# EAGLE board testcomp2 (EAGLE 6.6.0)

Size 100 x 80 mm. Coordinates in mm from the lower left corner, seen from the top.
Outline: 0,0 100,0 100,80 0,80 0,0
Copper layers (1*16): Top 0.035mm / dielectric 1.5mm / Bottom 0.035mm
Design rules "Fusion_eagle_rule_v1.1": minimum track width 6mil, minimum drill 12mil, track to track 6mil, track to pad 6mil, pad to pad 6mil, via to via 6mil, smd to smd 0mil, copper to edge 10mil, drill to drill 10mil, minimum pad ring 10mil, minimum via ring 6mil, stop-mask expansion 2mil, vias tented up to drill 100mil, thermal gap 10mil

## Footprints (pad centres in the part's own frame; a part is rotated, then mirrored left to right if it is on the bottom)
C0805 = smd 1.3 x 1.5: 1 -0.95,0; 2 0.95,0
SOT23 = smd 1 x 1.4: 1 -0.95,-1.1; 2 0.95,-1.1; 3 0,1.354
R0805 = smd 1.3 x 1.5: 1 -0.95,0; 2 0.95,0

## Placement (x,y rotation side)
C1  100nF  [C0805]  6.44,10.71 270 top
C2  100nF  [C0805]  5.56,6.29 90 top
C3  100nF  [C0805]  13.56,6.29 90 top
C4  100nF  [C0805]  14.44,10.71 270 top
C5  100nF  [C0805]  21.56,6.29 90 top
C6  100nF  [C0805]  22.44,10.71 270 top
C7  100nF  [C0805]  29.56,6.29 90 top
C8  100nF  [C0805]  30.44,10.71 270 top
C9  100nF  [C0805]  37.56,6.29 90 top
C10  100nF  [C0805]  38.44,10.71 270 top
C11  100nF  [C0805]  45.56,6.29 90 top
C12  100nF  [C0805]  46.44,10.71 270 top
C13  100nF  [C0805]  53.56,6.29 90 top
C14  100nF  [C0805]  54.44,10.71 270 top
C15  100nF  [C0805]  61.56,6.29 90 top
C16  100nF  [C0805]  62.44,10.71 270 top
C17  100nF  [C0805]  69.56,6.29 90 top
C18  100nF  [C0805]  70.44,10.71 270 top
C19  100nF  [C0805]  77.56,6.29 90 top
C20  100nF  [C0805]  78.44,10.71 270 top
C21  100nF  [C0805]  85.56,6.29 90 top
C22  100nF  [C0805]  86.44,10.71 270 top
C23  100nF  [C0805]  93.56,6.29 90 top
C24  100nF  [C0805]  94.44,10.71 270 top
C25  100nF  [C0805]  5.56,15.29 90 top
C26  100nF  [C0805]  6.44,19.71 270 top
C27  100nF  [C0805]  13.56,15.29 90 top
C28  100nF  [C0805]  14.44,19.71 270 top
C29  100nF  [C0805]  21.56,15.29 90 top
C30  100nF  [C0805]  22.44,19.71 270 top
C31  100nF  [C0805]  29.56,15.29 90 top
C32  100nF  [C0805]  30.44,19.71 270 top
C33  100nF  [C0805]  37.56,15.29 90 top
C34  100nF  [C0805]  38.44,19.71 270 top
C35  100nF  [C0805]  45.56,15.29 90 top
C36  100nF  [C0805]  46.44,19.71 270 top
C37  100nF  [C0805]  53.56,15.29 90 top
C38  100nF  [C0805]  54.44,19.71 270 top
C39  100nF  [C0805]  61.56,15.29 90 top
C40  100nF  [C0805]  62.44,19.71 270 top
C41  100nF  [C0805]  69.56,15.29 90 top
C42  100nF  [C0805]  70.44,19.71 270 top
C43  100nF  [C0805]  77.56,15.29 90 top
C44  100nF  [C0805]  78.44,19.71 270 top
C45  100nF  [C0805]  85.56,15.29 90 top
C46  100nF  [C0805]  86.44,19.71 270 top
C47  100nF  [C0805]  93.56,15.29 90 top
C48  100nF  [C0805]  94.44,19.71 270 top
C49  100nF  [C0805]  5.56,24.29 90 top
C50  100nF  [C0805]  6.44,28.71 270 top
C51  100nF  [C0805]  13.56,24.29 90 top
C52  100nF  [C0805]  14.44,28.71 270 top
C53  100nF  [C0805]  21.56,24.29 90 top
C54  100nF  [C0805]  22.44,28.71 270 top
C55  100nF  [C0805]  29.56,24.29 90 top
C56  100nF  [C0805]  30.44,28.71 270 top
C57  100nF  [C0805]  37.56,24.29 90 top
C58  100nF  [C0805]  38.44,28.71 270 top
C59  100nF  [C0805]  45.56,24.29 90 top
C60  100nF  [C0805]  46.44,28.71 270 top
C61  100nF  [C0805]  53.56,24.29 90 top
C62  100nF  [C0805]  54.44,28.71 270 top
C63  100nF  [C0805]  61.56,24.29 90 top
C64  100nF  [C0805]  62.44,28.71 270 top
C65  100nF  [C0805]  69.56,24.29 90 top
C66  100nF  [C0805]  70.44,28.71 270 top
C67  100nF  [C0805]  77.56,24.29 90 top
C68  100nF  [C0805]  78.44,28.71 270 top
C69  100nF  [C0805]  85.56,24.29 90 top
C70  100nF  [C0805]  86.44,28.71 270 top
C71  100nF  [C0805]  93.56,24.29 90 top
C72  100nF  [C0805]  94.44,28.71 270 top
C73  100nF  [C0805]  5.56,33.29 90 top
C74  100nF  [C0805]  6.44,37.71 270 top
C75  100nF  [C0805]  13.56,33.29 90 top
C76  100nF  [C0805]  14.44,37.71 270 top
C77  100nF  [C0805]  21.56,33.29 90 top
C78  100nF  [C0805]  22.44,37.71 270 top
C79  100nF  [C0805]  29.56,33.29 90 top
C80  100nF  [C0805]  30.44,37.71 270 top
C81  100nF  [C0805]  37.56,33.29 90 top
C82  100nF  [C0805]  38.44,37.71 270 top
C83  100nF  [C0805]  45.56,33.29 90 top
C84  100nF  [C0805]  46.44,37.71 270 top
C85  100nF  [C0805]  53.56,33.29 90 top
C86  100nF  [C0805]  54.44,37.71 270 top
C87  100nF  [C0805]  61.56,33.29 90 top
C88  100nF  [C0805]  62.44,37.71 270 top
C89  100nF  [C0805]  69.56,33.29 90 top
C90  100nF  [C0805]  70.44,37.71 270 top
C91  100nF  [C0805]  77.56,33.29 90 top
C92  100nF  [C0805]  78.44,37.71 270 top
C93  100nF  [C0805]  85.56,33.29 90 top
C94  100nF  [C0805]  86.44,37.71 270 top
C95  100nF  [C0805]  93.56,33.29 90 top
C96  100nF  [C0805]  94.44,37.71 270 top
C97  100nF  [C0805]  5.56,42.29 90 top
C98  100nF  [C0805]  6.44,46.71 270 top
C99  100nF  [C0805]  13.56,42.29 90 top
C100  100nF  [C0805]  14.44,46.71 270 top
C101  100nF  [C0805]  21.56,42.29 90 top
C102  100nF  [C0805]  22.44,46.71 270 top
C103  100nF  [C0805]  29.56,42.29 90 top
C104  100nF  [C0805]  30.44,46.71 270 top
C105  100nF  [C0805]  37.56,42.29 90 top
C106  100nF  [C0805]  38.44,46.71 270 top
C107  100nF  [C0805]  45.56,42.29 90 top
C108  100nF  [C0805]  46.44,46.71 270 top
C109  100nF  [C0805]  53.56,42.29 90 top
C110  100nF  [C0805]  54.44,46.71 270 top
C111  100nF  [C0805]  61.56,42.29 90 top
C112  100nF  [C0805]  62.44,46.71 270 top
C113  100nF  [C0805]  69.56,42.29 90 top
C114  100nF  [C0805]  70.44,46.71 270 top
C115  100nF  [C0805]  77.56,42.29 90 top
C116  100nF  [C0805]  78.44,46.71 270 top
C117  100nF  [C0805]  85.56,42.29 90 top
C118  100nF  [C0805]  86.44,46.71 270 top
C119  100nF  [C0805]  93.56,42.29 90 top
C120  100nF  [C0805]  94.44,46.71 270 top
C121  100nF  [C0805]  5.56,51.29 90 top
C122  100nF  [C0805]  6.44,55.71 270 top
C123  100nF  [C0805]  13.56,51.29 90 top
C124  100nF  [C0805]  14.44,55.71 270 top
C125  100nF  [C0805]  21.56,51.29 90 top
C126  100nF  [C0805]  22.44,55.71 270 top
C127  100nF  [C0805]  29.56,51.29 90 top
C128  100nF  [C0805]  30.44,55.71 270 top
C129  100nF  [C0805]  37.56,51.29 90 top
C130  100nF  [C0805]  38.44,55.71 270 top
C131  100nF  [C0805]  45.56,51.29 90 top
C132  100nF  [C0805]  46.44,55.71 270 top
C133  100nF  [C0805]  53.56,51.29 90 top
C134  100nF  [C0805]  54.44,55.71 270 top
C135  100nF  [C0805]  61.56,51.29 90 top
C136  100nF  [C0805]  62.44,55.71 270 top
C137  100nF  [C0805]  69.56,51.29 90 top
C138  100nF  [C0805]  70.44,55.71 270 top
C139  100nF  [C0805]  77.56,51.29 90 top
C140  100nF  [C0805]  78.44,55.71 270 top
C141  100nF  [C0805]  85.56,51.29 90 top
C142  100nF  [C0805]  86.44,55.71 270 top
C143  100nF  [C0805]  93.56,51.29 90 top
C144  100nF  [C0805]  94.44,55.71 270 top
C145  100nF  [C0805]  5.56,60.29 90 top
C146  100nF  [C0805]  6.44,64.71 270 top
C147  100nF  [C0805]  13.56,60.29 90 top
C148  100nF  [C0805]  14.44,64.71 270 top
C149  100nF  [C0805]  21.56,60.29 90 top
C150  100nF  [C0805]  22.44,64.71 270 top
C151  100nF  [C0805]  29.56,60.29 90 top
C152  100nF  [C0805]  30.44,64.71 270 top
C153  100nF  [C0805]  37.56,60.29 90 top
C154  100nF  [C0805]  38.44,64.71 270 top
C155  100nF  [C0805]  45.56,60.29 90 top
C156  100nF  [C0805]  46.44,64.71 270 top
C157  100nF  [C0805]  53.56,60.29 90 top
C158  100nF  [C0805]  54.44,64.71 270 top
C159  100nF  [C0805]  61.56,60.29 90 top
C160  100nF  [C0805]  62.44,64.71 270 top
C161  100nF  [C0805]  69.56,60.29 90 top
C162  100nF  [C0805]  70.44,64.71 270 top
C163  100nF  [C0805]  77.56,60.29 90 top
C164  100nF  [C0805]  78.44,64.71 270 top
C165  100nF  [C0805]  85.56,60.29 90 top
C166  100nF  [C0805]  86.44,64.71 270 top
C167  100nF  [C0805]  93.56,60.29 90 top
C168  100nF  [C0805]  94.44,64.71 270 top
C169  100nF  [C0805]  5.56,69.29 90 top
C170  100nF  [C0805]  6.44,73.71 270 top
C171  100nF  [C0805]  13.56,69.29 90 top
C172  100nF  [C0805]  14.44,73.71 270 top
C173  100nF  [C0805]  21.56,69.29 90 top
C174  100nF  [C0805]  22.44,73.71 270 top
C175  100nF  [C0805]  29.56,69.29 90 top
C176  100nF  [C0805]  30.44,73.71 270 top
C177  100nF  [C0805]  37.56,69.29 90 top
C178  100nF  [C0805]  38.44,73.71 270 top
C179  100nF  [C0805]  45.56,69.29 90 top
C180  100nF  [C0805]  46.44,73.71 270 top
C181  100nF  [C0805]  53.56,69.29 90 top
C182  100nF  [C0805]  54.44,73.71 270 top
C183  100nF  [C0805]  61.56,69.29 90 top
C184  100nF  [C0805]  62.44,73.71 270 top
C185  100nF  [C0805]  69.56,69.29 90 top
C186  100nF  [C0805]  70.44,73.71 270 top
C187  100nF  [C0805]  77.56,69.29 90 top
C188  100nF  [C0805]  78.44,73.71 270 top
C189  100nF  [C0805]  85.56,69.29 90 top
C190  100nF  [C0805]  86.44,73.71 270 top
C191  100nF  [C0805]  93.56,69.29 90 top
C192  100nF  [C0805]  94.44,73.71 270 top
D1  BAT54C  [SOT23]  3.78,10.35 0 top
D2  BAT54C  [SOT23]  8.22,6.65 180 top
D3  BAT54C  [SOT23]  11.78,10.35 0 top
D4  BAT54C  [SOT23]  16.22,6.65 180 top
D5  BAT54C  [SOT23]  19.78,10.35 0 top
D6  BAT54C  [SOT23]  24.22,6.65 180 top
D7  BAT54C  [SOT23]  27.78,10.35 0 top
D8  BAT54C  [SOT23]  32.22,6.65 180 top
D9  BAT54C  [SOT23]  35.78,10.35 0 top
D10  BAT54C  [SOT23]  40.22,6.65 180 top
D11  BAT54C  [SOT23]  43.78,10.35 0 top
D12  BAT54C  [SOT23]  48.22,6.65 180 top
D13  BAT54C  [SOT23]  51.78,10.35 0 top
D14  BAT54C  [SOT23]  56.22,6.65 180 top
D15  BAT54C  [SOT23]  59.78,10.35 0 top
D16  BAT54C  [SOT23]  64.22,6.65 180 top
D17  BAT54C  [SOT23]  67.78,10.35 0 top
D18  BAT54C  [SOT23]  72.22,6.65 180 top
D19  BAT54C  [SOT23]  75.78,10.35 0 top
D20  BAT54C  [SOT23]  80.22,6.65 180 top
D21  BAT54C  [SOT23]  83.78,10.35 0 top
D22  BAT54C  [SOT23]  88.22,6.65 180 top
D23  BAT54C  [SOT23]  91.78,10.35 0 top
D24  BAT54C  [SOT23]  96.22,6.65 180 top
D25  BAT54C  [SOT23]  3.78,19.35 0 top
D26  BAT54C  [SOT23]  8.22,15.65 180 top
D27  BAT54C  [SOT23]  11.78,19.35 0 top
D28  BAT54C  [SOT23]  16.22,15.65 180 top
D29  BAT54C  [SOT23]  19.78,19.35 0 top
D30  BAT54C  [SOT23]  24.22,15.65 180 top
D31  BAT54C  [SOT23]  27.78,19.35 0 top
D32  BAT54C  [SOT23]  32.22,15.65 180 top
D33  BAT54C  [SOT23]  35.78,19.35 0 top
D34  BAT54C  [SOT23]  40.22,15.65 180 top
D35  BAT54C  [SOT23]  43.78,19.35 0 top
D36  BAT54C  [SOT23]  48.22,15.65 180 top
D37  BAT54C  [SOT23]  51.78,19.35 0 top
D38  BAT54C  [SOT23]  56.22,15.65 180 top
D39  BAT54C  [SOT23]  59.78,19.35 0 top
D40  BAT54C  [SOT23]  64.22,15.65 180 top
D41  BAT54C  [SOT23]  67.78,19.35 0 top
D42  BAT54C  [SOT23]  72.22,15.65 180 top
D43  BAT54C  [SOT23]  75.78,19.35 0 top
D44  BAT54C  [SOT23]  80.22,15.65 180 top
D45  BAT54C  [SOT23]  83.78,19.35 0 top
D46  BAT54C  [SOT23]  88.22,15.65 180 top
D47  BAT54C  [SOT23]  91.78,19.35 0 top
D48  BAT54C  [SOT23]  96.22,15.65 180 top
D49  BAT54C  [SOT23]  3.78,28.35 0 top
D50  BAT54C  [SOT23]  8.22,24.65 180 top
D51  BAT54C  [SOT23]  11.78,28.35 0 top
D52  BAT54C  [SOT23]  16.22,24.65 180 top
D53  BAT54C  [SOT23]  19.78,28.35 0 top
D54  BAT54C  [SOT23]  24.22,24.65 180 top
D55  BAT54C  [SOT23]  27.78,28.35 0 top
D56  BAT54C  [SOT23]  32.22,24.65 180 top
D57  BAT54C  [SOT23]  35.78,28.35 0 top
D58  BAT54C  [SOT23]  40.22,24.65 180 top
D59  BAT54C  [SOT23]  43.78,28.35 0 top
D60  BAT54C  [SOT23]  48.22,24.65 180 top
D61  BAT54C  [SOT23]  51.78,28.35 0 top
D62  BAT54C  [SOT23]  56.22,24.65 180 top
D63  BAT54C  [SOT23]  59.78,28.35 0 top
D64  BAT54C  [SOT23]  64.22,24.65 180 top
D65  BAT54C  [SOT23]  67.78,28.35 0 top
D66  BAT54C  [SOT23]  72.22,24.65 180 top
D67  BAT54C  [SOT23]  75.78,28.35 0 top
D68  BAT54C  [SOT23]  80.22,24.65 180 top
D69  BAT54C  [SOT23]  83.78,28.35 0 top
D70  BAT54C  [SOT23]  88.22,24.65 180 top
D71  BAT54C  [SOT23]  91.78,28.35 0 top
D72  BAT54C  [SOT23]  96.22,24.65 180 top
D73  BAT54C  [SOT23]  3.78,37.35 0 top
D74  BAT54C  [SOT23]  8.22,33.65 180 top
D75  BAT54C  [SOT23]  11.78,37.35 0 top
D76  BAT54C  [SOT23]  16.22,33.65 180 top
D77  BAT54C  [SOT23]  19.78,37.35 0 top
D78  BAT54C  [SOT23]  24.22,33.65 180 top
D79  BAT54C  [SOT23]  27.78,37.35 0 top
D80  BAT54C  [SOT23]  32.22,33.65 180 top
D81  BAT54C  [SOT23]  35.78,37.35 0 top
D82  BAT54C  [SOT23]  40.22,33.65 180 top
D83  BAT54C  [SOT23]  43.78,37.35 0 top
D84  BAT54C  [SOT23]  48.22,33.65 180 top
D85  BAT54C  [SOT23]  51.78,37.35 0 top
D86  BAT54C  [SOT23]  56.22,33.65 180 top
D87  BAT54C  [SOT23]  59.78,37.35 0 top
D88  BAT54C  [SOT23]  64.22,33.65 180 top
D89  BAT54C  [SOT23]  67.78,37.35 0 top
D90  BAT54C  [SOT23]  72.22,33.65 180 top
D91  BAT54C  [SOT23]  75.78,37.35 0 top
D92  BAT54C  [SOT23]  80.22,33.65 180 top
D93  BAT54C  [SOT23]  83.78,37.35 0 top
D94  BAT54C  [SOT23]  88.22,33.65 180 top
D95  BAT54C  [SOT23]  91.78,37.35 0 top
D96  BAT54C  [SOT23]  96.22,33.65 180 top
D97  BAT54C  [SOT23]  3.78,46.35 0 top
D98  BAT54C  [SOT23]  8.22,42.65 180 top
D99  BAT54C  [SOT23]  11.78,46.35 0 top
D100  BAT54C  [SOT23]  16.22,42.65 180 top
D101  BAT54C  [SOT23]  19.78,46.35 0 top
D102  BAT54C  [SOT23]  24.22,42.65 180 top
D103  BAT54C  [SOT23]  27.78,46.35 0 top
D104  BAT54C  [SOT23]  32.22,42.65 180 top
D105  BAT54C  [SOT23]  35.78,46.35 0 top
D106  BAT54C  [SOT23]  40.22,42.65 180 top
D107  BAT54C  [SOT23]  43.78,46.35 0 top
D108  BAT54C  [SOT23]  48.22,42.65 180 top
D109  BAT54C  [SOT23]  51.78,46.35 0 top
D110  BAT54C  [SOT23]  56.22,42.65 180 top
D111  BAT54C  [SOT23]  59.78,46.35 0 top
D112  BAT54C  [SOT23]  64.22,42.65 180 top
D113  BAT54C  [SOT23]  67.78,46.35 0 top
D114  BAT54C  [SOT23]  72.22,42.65 180 top
D115  BAT54C  [SOT23]  75.78,46.35 0 top
D116  BAT54C  [SOT23]  80.22,42.65 180 top
D117  BAT54C  [SOT23]  83.78,46.35 0 top
D118  BAT54C  [SOT23]  88.22,42.65 180 top
D119  BAT54C  [SOT23]  91.78,46.35 0 top
D120  BAT54C  [SOT23]  96.22,42.65 180 top
D121  BAT54C  [SOT23]  3.78,55.35 0 top
D122  BAT54C  [SOT23]  8.22,51.65 180 top
D123  BAT54C  [SOT23]  11.78,55.35 0 top
D124  BAT54C  [SOT23]  16.22,51.65 180 top
D125  BAT54C  [SOT23]  19.78,55.35 0 top
D126  BAT54C  [SOT23]  24.22,51.65 180 top
D127  BAT54C  [SOT23]  27.78,55.35 0 top
D128  BAT54C  [SOT23]  32.22,51.65 180 top
D129  BAT54C  [SOT23]  35.78,55.35 0 top
D130  BAT54C  [SOT23]  40.22,51.65 180 top
D131  BAT54C  [SOT23]  43.78,55.35 0 top
D132  BAT54C  [SOT23]  48.22,51.65 180 top
D133  BAT54C  [SOT23]  51.78,55.35 0 top
D134  BAT54C  [SOT23]  56.22,51.65 180 top
D135  BAT54C  [SOT23]  59.78,55.35 0 top
D136  BAT54C  [SOT23]  64.22,51.65 180 top
D137  BAT54C  [SOT23]  67.78,55.35 0 top
D138  BAT54C  [SOT23]  72.22,51.65 180 top
D139  BAT54C  [SOT23]  75.78,55.35 0 top
D140  BAT54C  [SOT23]  80.22,51.65 180 top
D141  BAT54C  [SOT23]  83.78,55.35 0 top
D142  BAT54C  [SOT23]  88.22,51.65 180 top
D143  BAT54C  [SOT23]  91.78,55.35 0 top
D144  BAT54C  [SOT23]  96.22,51.65 180 top
D145  BAT54C  [SOT23]  3.78,64.35 0 top
D146  BAT54C  [SOT23]  8.22,60.65 180 top
D147  BAT54C  [SOT23]  11.78,64.35 0 top
D148  BAT54C  [SOT23]  16.22,60.65 180 top
D149  BAT54C  [SOT23]  19.78,64.35 0 top
D150  BAT54C  [SOT23]  24.22,60.65 180 top
D151  BAT54C  [SOT23]  27.78,64.35 0 top
D152  BAT54C  [SOT23]  32.22,60.65 180 top
D153  BAT54C  [SOT23]  35.78,64.35 0 top
D154  BAT54C  [SOT23]  40.22,60.65 180 top
D155  BAT54C  [SOT23]  43.78,64.35 0 top
D156  BAT54C  [SOT23]  48.22,60.65 180 top
D157  BAT54C  [SOT23]  51.78,64.35 0 top
D158  BAT54C  [SOT23]  56.22,60.65 180 top
D159  BAT54C  [SOT23]  59.78,64.35 0 top
D160  BAT54C  [SOT23]  64.22,60.65 180 top
D161  BAT54C  [SOT23]  67.78,64.35 0 top
D162  BAT54C  [SOT23]  72.22,60.65 180 top
D163  BAT54C  [SOT23]  75.78,64.35 0 top
D164  BAT54C  [SOT23]  80.22,60.65 180 top
D165  BAT54C  [SOT23]  83.78,64.35 0 top
D166  BAT54C  [SOT23]  88.22,60.65 180 top
D167  BAT54C  [SOT23]  91.78,64.35 0 top
D168  BAT54C  [SOT23]  96.22,60.65 180 top
D169  BAT54C  [SOT23]  3.78,73.35 0 top
D170  BAT54C  [SOT23]  8.22,69.65 180 top
D171  BAT54C  [SOT23]  11.78,73.35 0 top
D172  BAT54C  [SOT23]  16.22,69.65 180 top
D173  BAT54C  [SOT23]  19.78,73.35 0 top
D174  BAT54C  [SOT23]  24.22,69.65 180 top
D175  BAT54C  [SOT23]  27.78,73.35 0 top
D176  BAT54C  [SOT23]  32.22,69.65 180 top
D177  BAT54C  [SOT23]  35.78,73.35 0 top
D178  BAT54C  [SOT23]  40.22,69.65 180 top
D179  BAT54C  [SOT23]  43.78,73.35 0 top
D180  BAT54C  [SOT23]  48.22,69.65 180 top
D181  BAT54C  [SOT23]  51.78,73.35 0 top
D182  BAT54C  [SOT23]  56.22,69.65 180 top
D183  BAT54C  [SOT23]  59.78,73.35 0 top
D184  BAT54C  [SOT23]  64.22,69.65 180 top
D185  BAT54C  [SOT23]  67.78,73.35 0 top
D186  BAT54C  [SOT23]  72.22,69.65 180 top
D187  BAT54C  [SOT23]  75.78,73.35 0 top
D188  BAT54C  [SOT23]  80.22,69.65 180 top
D189  BAT54C  [SOT23]  83.78,73.35 0 top
D190  BAT54C  [SOT23]  88.22,69.65 180 top
D191  BAT54C  [SOT23]  91.78,73.35 0 top
D192  BAT54C  [SOT23]  96.22,69.65 180 top
R1  10k  [R0805]  3.27,6.29 90 top
R2  10k  [R0805]  8.73,10.71 270 top
R3  10k  [R0805]  11.27,6.29 90 top
R4  10k  [R0805]  16.73,10.71 270 top
R5  10k  [R0805]  19.27,6.29 90 top
R6  10k  [R0805]  24.73,10.71 270 top
R7  10k  [R0805]  27.27,6.29 90 top
R8  10k  [R0805]  32.73,10.71 270 top
R9  10k  [R0805]  35.27,6.29 90 top
R10  10k  [R0805]  40.73,10.71 270 top
R11  10k  [R0805]  43.27,6.29 90 top
R12  10k  [R0805]  48.73,10.71 270 top
R13  10k  [R0805]  51.27,6.29 90 top
R14  10k  [R0805]  56.73,10.71 270 top
R15  10k  [R0805]  59.27,6.29 90 top
R16  10k  [R0805]  64.73,10.71 270 top
R17  10k  [R0805]  67.27,6.29 90 top
R18  10k  [R0805]  72.73,10.71 270 top
R19  10k  [R0805]  75.27,6.29 90 top
R20  10k  [R0805]  80.73,10.71 270 top
R21  10k  [R0805]  83.27,6.29 90 top
R22  10k  [R0805]  88.73,10.71 270 top
R23  10k  [R0805]  91.27,6.29 90 top
R24  10k  [R0805]  96.73,10.71 270 top
R25  10k  [R0805]  3.27,15.29 90 top
R26  10k  [R0805]  8.73,19.71 270 top
R27  10k  [R0805]  11.27,15.29 90 top
R28  10k  [R0805]  16.73,19.71 270 top
R29  10k  [R0805]  19.27,15.29 90 top
R30  10k  [R0805]  24.73,19.71 270 top
R31  10k  [R0805]  27.27,15.29 90 top
R32  10k  [R0805]  32.73,19.71 270 top
R33  10k  [R0805]  35.27,15.29 90 top
R34  10k  [R0805]  40.73,19.71 270 top
R35  10k  [R0805]  43.27,15.29 90 top
R36  10k  [R0805]  48.73,19.71 270 top
R37  10k  [R0805]  51.27,15.29 90 top
R38  10k  [R0805]  56.73,19.71 270 top
R39  10k  [R0805]  59.27,15.29 90 top
R40  10k  [R0805]  64.73,19.71 270 top
R41  10k  [R0805]  67.27,15.29 90 top
R42  10k  [R0805]  72.73,19.71 270 top
R43  10k  [R0805]  75.27,15.29 90 top
R44  10k  [R0805]  80.73,19.71 270 top
R45  10k  [R0805]  83.27,15.29 90 top
R46  10k  [R0805]  88.73,19.71 270 top
R47  10k  [R0805]  91.27,15.29 90 top
R48  10k  [R0805]  96.73,19.71 270 top
R49  10k  [R0805]  3.27,24.29 90 top
R50  10k  [R0805]  8.73,28.71 270 top
R51  10k  [R0805]  11.27,24.29 90 top
R52  10k  [R0805]  16.73,28.71 270 top
R53  10k  [R0805]  19.27,24.29 90 top
R54  10k  [R0805]  24.73,28.71 270 top
R55  10k  [R0805]  27.27,24.29 90 top
R56  10k  [R0805]  32.73,28.71 270 top
R57  10k  [R0805]  35.27,24.29 90 top
R58  10k  [R0805]  40.73,28.71 270 top
R59  10k  [R0805]  43.27,24.29 90 top
R60  10k  [R0805]  48.73,28.71 270 top
R61  10k  [R0805]  51.27,24.29 90 top
R62  10k  [R0805]  56.73,28.71 270 top
R63  10k  [R0805]  59.27,24.29 90 top
R64  10k  [R0805]  64.73,28.71 270 top
R65  10k  [R0805]  67.27,24.29 90 top
R66  10k  [R0805]  72.73,28.71 270 top
R67  10k  [R0805]  75.27,24.29 90 top
R68  10k  [R0805]  80.73,28.71 270 top
R69  10k  [R0805]  83.27,24.29 90 top
R70  10k  [R0805]  88.73,28.71 270 top
R71  10k  [R0805]  91.27,24.29 90 top
R72  10k  [R0805]  96.73,28.71 270 top
R73  10k  [R0805]  3.27,33.29 90 top
R74  10k  [R0805]  8.73,37.71 270 top
R75  10k  [R0805]  11.27,33.29 90 top
R76  10k  [R0805]  16.73,37.71 270 top
R77  10k  [R0805]  19.27,33.29 90 top
R78  10k  [R0805]  24.73,37.71 270 top
R79  10k  [R0805]  27.27,33.29 90 top
R80  10k  [R0805]  32.73,37.71 270 top
R81  10k  [R0805]  35.27,33.29 90 top
R82  10k  [R0805]  40.73,37.71 270 top
R83  10k  [R0805]  43.27,33.29 90 top
R84  10k  [R0805]  48.73,37.71 270 top
R85  10k  [R0805]  51.27,33.29 90 top
R86  10k  [R0805]  56.73,37.71 270 top
R87  10k  [R0805]  59.27,33.29 90 top
R88  10k  [R0805]  64.73,37.71 270 top
R89  10k  [R0805]  67.27,33.29 90 top
R90  10k  [R0805]  72.73,37.71 270 top
R91  10k  [R0805]  75.27,33.29 90 top
R92  10k  [R0805]  80.73,37.71 270 top
R93  10k  [R0805]  83.27,33.29 90 top
R94  10k  [R0805]  88.73,37.71 270 top
R95  10k  [R0805]  91.27,33.29 90 top
R96  10k  [R0805]  96.73,37.71 270 top
R97  10k  [R0805]  3.27,42.29 90 top
R98  10k  [R0805]  8.73,46.71 270 top
R99  10k  [R0805]  11.27,42.29 90 top
R100  10k  [R0805]  16.73,46.71 270 top
R101  10k  [R0805]  19.27,42.29 90 top
R102  10k  [R0805]  24.73,46.71 270 top
R103  10k  [R0805]  27.27,42.29 90 top
R104  10k  [R0805]  32.73,46.71 270 top
R105  10k  [R0805]  35.27,42.29 90 top
R106  10k  [R0805]  40.73,46.71 270 top
R107  10k  [R0805]  43.27,42.29 90 top
R108  10k  [R0805]  48.73,46.71 270 top
R109  10k  [R0805]  51.27,42.29 90 top
R110  10k  [R0805]  56.73,46.71 270 top
R111  10k  [R0805]  59.27,42.29 90 top
R112  10k  [R0805]  64.73,46.71 270 top
R113  10k  [R0805]  67.27,42.29 90 top
R114  10k  [R0805]  72.73,46.71 270 top
R115  10k  [R0805]  75.27,42.29 90 top
R116  10k  [R0805]  80.73,46.71 270 top
R117  10k  [R0805]  83.27,42.29 90 top
R118  10k  [R0805]  88.73,46.71 270 top
R119  10k  [R0805]  91.27,42.29 90 top
R120  10k  [R0805]  96.73,46.71 270 top
R121  10k  [R0805]  3.27,51.29 90 top
R122  10k  [R0805]  8.73,55.71 270 top
R123  10k  [R0805]  11.27,51.29 90 top
R124  10k  [R0805]  16.73,55.71 270 top
R125  10k  [R0805]  19.27,51.29 90 top
R126  10k  [R0805]  24.73,55.71 270 top
R127  10k  [R0805]  27.27,51.29 90 top
R128  10k  [R0805]  32.73,55.71 270 top
R129  10k  [R0805]  35.27,51.29 90 top
R130  10k  [R0805]  40.73,55.71 270 top
R131  10k  [R0805]  43.27,51.29 90 top
R132  10k  [R0805]  48.73,55.71 270 top
R133  10k  [R0805]  51.27,51.29 90 top
R134  10k  [R0805]  56.73,55.71 270 top
R135  10k  [R0805]  59.27,51.29 90 top
R136  10k  [R0805]  64.73,55.71 270 top
R137  10k  [R0805]  67.27,51.29 90 top
R138  10k  [R0805]  72.73,55.71 270 top
R139  10k  [R0805]  75.27,51.29 90 top
R140  10k  [R0805]  80.73,55.71 270 top
R141  10k  [R0805]  83.27,51.29 90 top
R142  10k  [R0805]  88.73,55.71 270 top
R143  10k  [R0805]  91.27,51.29 90 top
R144  10k  [R0805]  96.73,55.71 270 top
R145  10k  [R0805]  3.27,60.29 90 top
R146  10k  [R0805]  8.73,64.71 270 top
R147  10k  [R0805]  11.27,60.29 90 top
R148  10k  [R0805]  16.73,64.71 270 top
R149  10k  [R0805]  19.27,60.29 90 top
R150  10k  [R0805]  24.73,64.71 270 top
R151  10k  [R0805]  27.27,60.29 90 top
R152  10k  [R0805]  32.73,64.71 270 top
R153  10k  [R0805]  35.27,60.29 90 top
R154  10k  [R0805]  40.73,64.71 270 top
R155  10k  [R0805]  43.27,60.29 90 top
R156  10k  [R0805]  48.73,64.71 270 top
R157  10k  [R0805]  51.27,60.29 90 top
R158  10k  [R0805]  56.73,64.71 270 top
R159  10k  [R0805]  59.27,60.29 90 top
R160  10k  [R0805]  64.73,64.71 270 top
R161  10k  [R0805]  67.27,60.29 90 top
R162  10k  [R0805]  72.73,64.71 270 top
R163  10k  [R0805]  75.27,60.29 90 top
R164  10k  [R0805]  80.73,64.71 270 top
R165  10k  [R0805]  83.27,60.29 90 top
R166  10k  [R0805]  88.73,64.71 270 top
R167  10k  [R0805]  91.27,60.29 90 top
R168  10k  [R0805]  96.73,64.71 270 top
R169  10k  [R0805]  3.27,69.29 90 top
R170  10k  [R0805]  8.73,73.71 270 top
R171  10k  [R0805]  11.27,69.29 90 top
R172  10k  [R0805]  16.73,73.71 270 top
R173  10k  [R0805]  19.27,69.29 90 top
R174  10k  [R0805]  24.73,73.71 270 top
R175  10k  [R0805]  27.27,69.29 90 top
R176  10k  [R0805]  32.73,73.71 270 top
R177  10k  [R0805]  35.27,69.29 90 top
R178  10k  [R0805]  40.73,73.71 270 top
R179  10k  [R0805]  43.27,69.29 90 top
R180  10k  [R0805]  48.73,73.71 270 top
R181  10k  [R0805]  51.27,69.29 90 top
R182  10k  [R0805]  56.73,73.71 270 top
R183  10k  [R0805]  59.27,69.29 90 top
R184  10k  [R0805]  64.73,73.71 270 top
R185  10k  [R0805]  67.27,69.29 90 top
R186  10k  [R0805]  72.73,73.71 270 top
R187  10k  [R0805]  75.27,69.29 90 top
R188  10k  [R0805]  80.73,73.71 270 top
R189  10k  [R0805]  83.27,69.29 90 top
R190  10k  [R0805]  88.73,73.71 270 top
R191  10k  [R0805]  91.27,69.29 90 top
R192  10k  [R0805]  96.73,73.71 270 top

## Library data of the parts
C1-C192 = rcl; LCSC: C476766
D1-D192 = hdr_altera; LCSC: C556168
R1-R192 = rcl; LCSC: C84376

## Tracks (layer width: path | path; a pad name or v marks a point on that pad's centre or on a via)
GND  (67 unrouted)
PGND  (74 unrouted)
